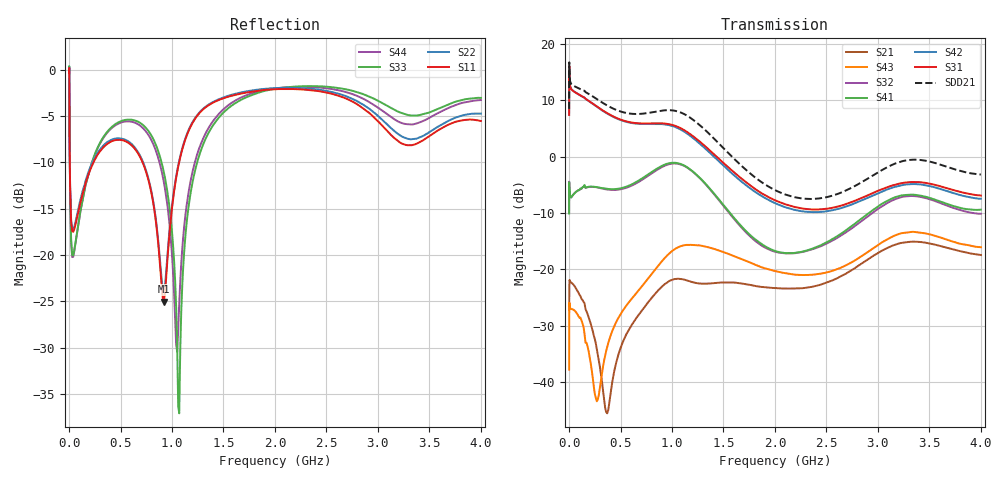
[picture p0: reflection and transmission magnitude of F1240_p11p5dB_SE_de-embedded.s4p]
! Integrated Device Technology
! Corporate Headquarters
! 6024 Silver Creek Valley Road
! San Jose, CA 95138  USA
! Phone:  1-408-284-8200
! Toll Free:  1-800-223-1366
! Webpage:  http://www.idt.com/
! Timing and RF Division
! 515 Groton Road, Suite 102
! Westford, MA 01886-6024
! Device:  F1240
! Description: Dual Intermediate Frequency Digital Variable Gain Amplifier
! Frequency:  10.0 -  500.00 MHz
! Package:  5x5 mm QFN Plastic Package: 32 pin
! Ports:  8 RF, 20 DC
!  Pin  1  = GA3 / Data  Pin 17  = RF OUT_B+
!  Pin  2  = GA4 / CLK  Pin 18  = RF OUT_B-
!  Pin  3  = GA5  Pin 19  = STBY_B
!  Pin  4  = VMODE  Pin 20  = Ground
!  Pin  5  = No Connect  Pin 21  = Ground
!  Pin  6  = GB5  Pin 22  = STB_A
!  Pin  7  = GB4  Pin 23  = RF OUT_A-  = Port 4
!  Pin  8  = GB3  Pin 24  = RF OUT_A+  = Port 3
!  Pin  9  = GB2  Pin 25  = GA0
!  Pin 10  = GB1  Pin 26  = ISET_A
!  Pin 11  = RF IN_B+  Pin 27  = VCC
!  Pin 12  = RF IN_B-  Pin 28  = Ground
!  Pin 13  = Ground  Pin 29  = RF IN_A-  = Port 2
!  Pin 14  = VCC  Pin 30  = RF IN_A+  = Port 1
!  Pin 15  = ISET_B  Pin 31  = GA1
!  Pin 16  = GB0  Pin 32  = GA2 / CSb
! Gain  = +19.5 dB
! State  = 1
! Voltage  = +5.00 V
! Current  = 85.292 mA (one channel only)
! Temperture  =  +25 C
! Test Date  =  2017-10-18
! Board  =  EB4031
! Data:  The device was measured on a custom evaluation board which has
!  individual transmission lines to the RF pins.  Data was collected
!  using a calibrated network analyzer.  The evaluation board was
!  de-embedded using Automatic Fixture Removal.
!  The reference plane is the edge of the package pin.
!  Only Channel A was measured.
!  This data is in single-ended operation.  If your needs are balanced
!  or differential S-parameters then this file needs to be used a
!  linear simulator.
! File Date:  2017-11-10  MJV
! Note:
!  Integrated Device Technology supplies this data as a sample of measured
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# Hz S dB R 100
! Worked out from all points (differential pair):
!   410 points, 500 kHz to 4 GHz, reference 100 ohm
!   strongest paths, dB at 500 kHz, 930 MHz, 1.96 GHz, 2.98 GHz, 4 GHz:
!     S31: 7.4, 5.9, -7.4, -6.2, -6.9
!     S42: 7.4, 5.7, -7.9, -6.7, -7.5
!     S41: -10.1, -1.4, -16.5, -9.1, -9.4
!     S32: -10.0, -1.6, -16.6, -9.5, -10.1
!     S43: -37.8, -18.0, -20.1, -16.0, -16.1
!     S21: -26.6, -22.6, -23.3, -17.3, -17.5
!   taken as a pair (ports 1,2 in; 3,4 out), SDD21 dB: 8.5, 8.2, -5.5, -3.0, -3.2
!   lowest |S11| = -25.0 dB at 920 MHz (marker M1), VSWR 1.12, Z = 110 + j5.97 ohm
!   |S11| at or under -10 dB: 7.52 MHz to 238 MHz (230.4 MHz wide, 188 % of centre); 713.7 MHz to 1.069 GHz (355.3 MHz wide, 39.9 % of centre)
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500000  -0.37 -5.8  -26.61 -2.0  -27.23 80.3  -59.45 69.1
        -26.59 -2.1  -0.37 -5.7  -58.87 69.1  -27.24 81.5
        7.42 -105.2  -10.04 69.9  -0.46 1.3  -37.84 -127.7
        -10.10 71.0  7.40 -104.0  -37.81 -127.3  -0.47 3.6
3000000  -3.39 -60.0  -22.70 9.7  -16.90 20.6  -43.42 66.8
         -22.69 9.8  -3.35 -60.0  -43.43 66.2  -16.91 20.8
         15.28 -177.8  -5.38 -9.9  -2.91 -55.8  -25.98 54.8
         -5.34 -9.8  15.28 -177.6  -25.94 54.8  -2.97 -55.5
2e8  -10.96 -129.8  -28.94 -83.9  -19.20 -50.4  -34.41 10.5
     -29.07 -82.5  -10.71 -131.0  -34.35 11.2  -19.22 -50.5
     9.81 109.7  -5.37 -40.8  -10.84 -92.2  -34.44 -105.7
     -5.32 -41.1  9.78 109.0  -35.56 -101.9  -10.86 -91.2
5.3e8  -7.66 -178.8  -33.52 -9.7  -20.50 -107.6  -28.50 -57.2
       -32.59 -13.8  -7.51 -180.0  -28.62 -55.4  -20.63 -107.8
       6.40 26.6  -5.67 -107.1  -5.47 -155.4  -28.64 19.6
       -5.48 -108.6  6.32 25.6  -27.13 13.3  -5.64 -155.2
9.2e8  -25.02 28.8  -22.66 -79.8  -18.25 169.8  -24.68 -149.1
       -22.78 -89.0  -23.96 28.0  -24.95 -143.3  -18.59 169.2
       5.90 -70.5  -1.68 160.2  -11.03 139.1  -19.30 -63.9
       -1.48 156.0  5.76 -72.3  -18.18 -71.8  -12.10 141.6
1.52e9  -3.02 -149.8  -21.80 142.4  -24.23 29.7  -26.44 74.6
        -22.33 145.4  -2.93 -149.6  -26.22 80.2  -25.21 29.5
        -1.45 126.7  -9.21 -21.6  -4.43 -137.1  -17.51 131.6
        -9.05 -27.0  -1.95 125.6  -17.08 127.9  -4.08 -140.1
4e9  -5.55 -153.3  -17.53 72.0  -20.91 -57.5  -20.53 -47.9
     -17.46 71.5  -4.75 -149.2  -22.27 -28.6  -23.39 -49.2
     -6.90 14.8  -10.15 -106.4  -3.06 -138.4  -16.24 87.4
     -9.41 -119.1  -7.48 23.4  -16.08 61.3  -3.29 -144.8
